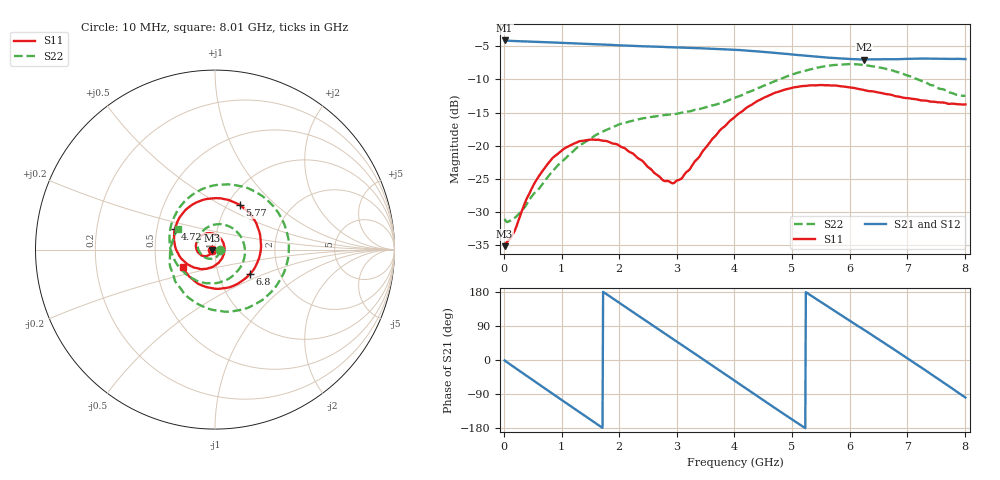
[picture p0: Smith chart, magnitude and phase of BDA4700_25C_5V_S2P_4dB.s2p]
!Agilent Technologies,E5071B,MY42404982,A.09.10
!Date: Mon Oct 20 13:27:54 2025
!Data & Calibration Information:
!Freq	S11:SOLT2(ON)	S21:SOLT2(ON)	S12:SOLT2(ON)	S22:SOLT2(ON)
# Hz S RI R 50
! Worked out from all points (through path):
!   801 points, 10 MHz to 8.01 GHz, reference 50 ohm
!   highest |S21| = -4.12 dB at 10 MHz (marker M1); lowest = -7.0 dB at 6.25 GHz (marker M2)
!   group delay of S21, straight-line fit = 283 ps
!   lowest |S11| = -35.1 dB at 10 MHz (marker M3), VSWR 1.04, Z = 48.3 - j0.126 ohm
!   |S11| at or under -10 dB: start of sweep to end of sweep
!   |S22| runs from -31.5 to -7.7 dB; largest |S21 - S12| = 0.0048
!   S11 on the Smith chart (normalised r, x): 10 MHz: 0.97, -0.00; 4.72 GHz: 0.62, +0.15; 5.77 GHz: 1.14, +0.62; 6.8 GHz: 1.41, -0.41; 8.01 GHz: 0.68, -0.14
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1e7  -0.0175 -0.0013  0.6221 -0.0133  0.622 -0.014  0.0281 -0.00261
3.3e8  -0.0252 -0.0231  0.5004 -0.3533  0.5001 -0.3538  0.0193 -0.0271
7.1e8  -0.058 -0.0363  0.1554 -0.5837  0.1552 -0.5844  -0.0199 -0.051
1.02e9  -0.0915 -0.0191  -0.1788 -0.5695  -0.1793 -0.5695  -0.0693 -0.0342
1.35e9  -0.1066 0.0233  -0.4628 -0.3642  -0.4628 -0.3644  -0.0978 0.0318
1.64e9  -0.0909 0.0642  -0.5758 -0.0824  -0.5759 -0.0825  -0.0698 0.1018
1.93e9  -0.0525 0.0893  -0.533 0.213  -0.5328 0.2136  0.0081 0.1406
2.32e9  0.00819 0.0805  -0.2664 0.4976  -0.2666 0.4982  0.1256 0.0957
2.68e9  0.0469 0.0366  0.0841 0.5514  0.0841 0.5517  0.1662 -0.0258
2.96e9  0.0511 -0.0132  0.3348 0.4389  0.3353 0.4383  0.1248 -0.1204
3.37e9  0.0112 -0.0799  0.5349 0.1006  0.5355 0.0995  -0.0123 -0.1877
3.68e9  -0.0545 -0.1071  0.5004 -0.1944  0.5006 -0.196  -0.129 -0.1586
4.01e9  -0.1395 -0.0894  0.3007 -0.4348  0.3011 -0.4344  -0.2204 -0.0665
4.36e9  -0.2119 -0.00921  -0.0121 -0.516  -0.0127 -0.5165  -0.2539 0.0817
4.72e9  -0.2235 0.117  -0.3109 -0.3927  -0.31 -0.3935  -0.1911 0.243
5.35e9  -0.0428 0.2823  -0.4626 0.0988  -0.463 0.0976  0.1347 0.3546
5.77e9  0.1366 0.2495  -0.2719 0.3682  -0.2711 0.369  0.3522 0.2056
6.25e9  0.2518 0.0798  0.0798 0.44  0.0845 0.4395  0.3916 -0.1074
6.68e9  0.2235 -0.0986  0.3582 0.27  0.3595 0.2695  0.2057 -0.3137
6.8e9  0.1925 -0.1378  0.4069 0.1908  0.4084 0.1889  0.1338 -0.3375
7.33e9  0.00959 -0.2188  0.3985 -0.2175  0.3987 -0.2191  -0.1695 -0.2476
8.01e9  -0.1808 -0.0972  -0.0715 -0.4448  -0.071 -0.4452  -0.2077 0.116
